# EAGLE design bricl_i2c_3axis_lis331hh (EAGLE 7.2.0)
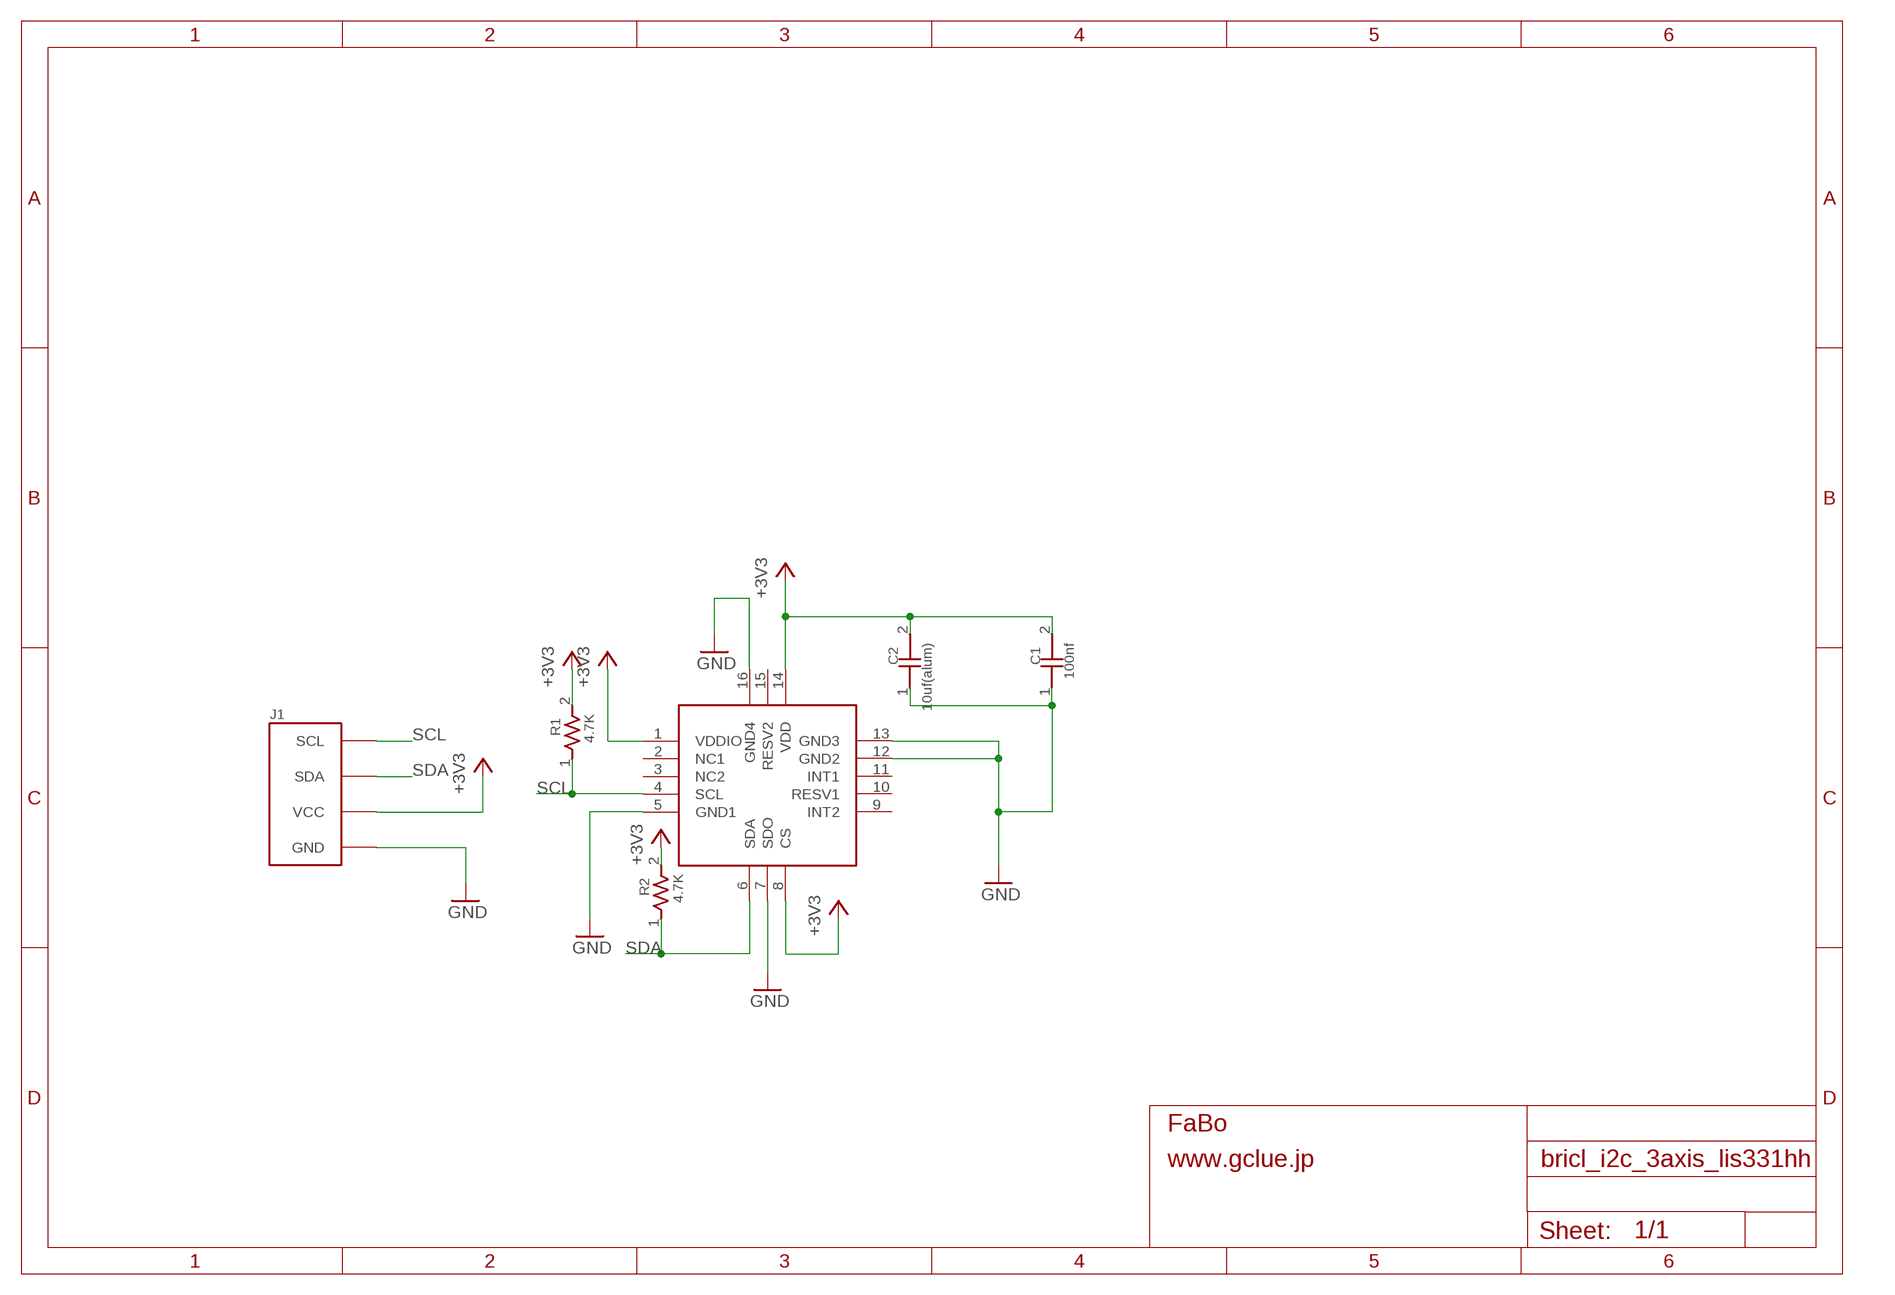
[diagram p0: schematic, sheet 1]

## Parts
C1  100nf  CAPACITOR0603  [0603]
C2  10uf(alum)  CAPACITOR0603  [0603]
J1  BRICK_I2C  [BRICK_I2C]
R1  4.7K  RESISTOR0603  [0603]
R2  4.7K  RESISTOR0603  [0603]
U$1  ST-LIS331HH  [ST-LIS331HH]

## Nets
+3V3: C1.2 C2.2 J1.VCC R1.2 R2.2 U$1.1(VDDIO) U$1.8(CS) U$1.14(VDD)
GND: C1.1 C2.1 J1.GND U$1.5(GND1) U$1.7(SDO) U$1.12(GND2) U$1.13(GND3) U$1.16(GND4)
SCL: J1.SCL R1.1 U$1.4(SCL)
SDA: J1.SDA R2.1 U$1.6(SDA)
Unconnected: U$1.2(NC1) U$1.3(NC2) U$1.9(INT2) U$1.10(RESV1) U$1.11(INT1) U$1.15(RESV2)

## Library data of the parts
C1 C2 = GClue-Capacitor:CAPACITOR
J1 = gclue:BRICK_I2C: FaBo Brick 4pin(I2C)
R1 R2 = GClue-Resistors:RESISTOR
U$1 = GClue-Mems:ST-LIS331HH

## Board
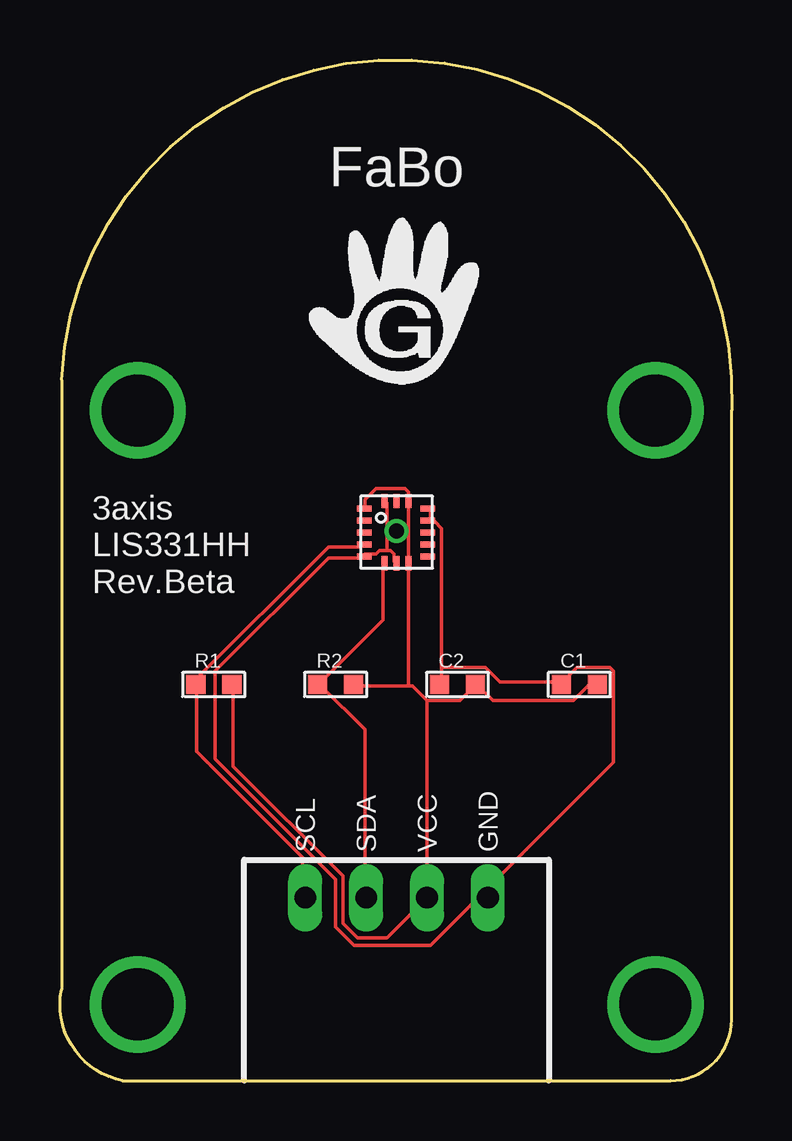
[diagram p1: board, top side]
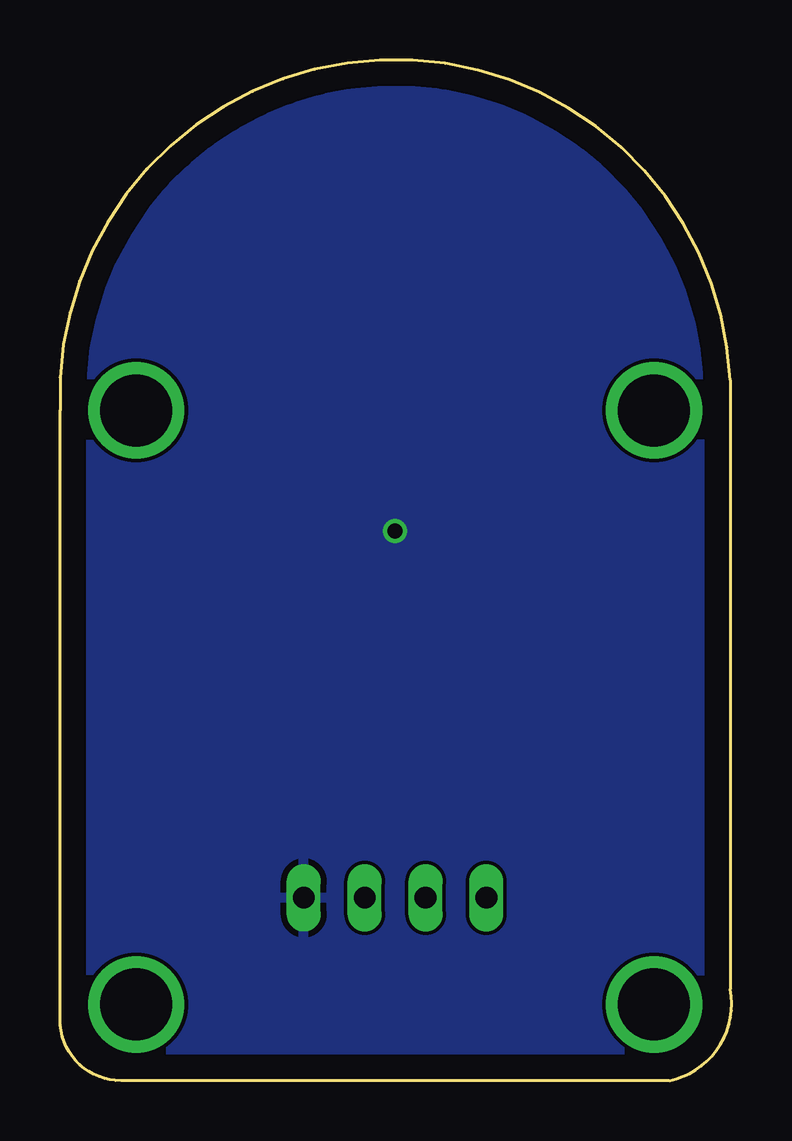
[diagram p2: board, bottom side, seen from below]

Size 28 x 42.55 mm. Coordinates in mm from the lower left corner, seen from the top.
Copper layers (1*16): Top 0.035mm / dielectric 1.5mm / Bottom 0.035mm
Design rules "default *": minimum track width 6mil, minimum drill 24mil, track to track 6mil, track to pad 6mil, pad to pad 6mil, via to via 6mil, smd to smd 6mil, copper to edge 40mil, drill to drill 8mil, minimum pad ring 10mil, minimum via ring 8mil, stop-mask expansion 4mil, vias tented up to drill 0mil, thermal gap 10mil

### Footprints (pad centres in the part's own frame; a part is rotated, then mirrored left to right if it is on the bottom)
0603 = smd 0.8 x 0.8: 1 -0.75,0; 2 0.75,0
BRICK_I2C = drill 0.9 long: GND 3.81,-12.7; SCL -3.81,-12.7; SDA -1.27,-12.7; VCC 1.27,-12.7 | drill 3 pad 3.81: P$5 -10.795,7.62; P$6 10.795,7.62; P$7 -10.795,-17.145; P$8 10.795,-17.145
ST-LIS331HH = smd 0.6 x 0.25: 1 -1.35,0.98; 2 -1.35,0.48; 3 -1.35,-0.02; 4 -1.35,-0.52; 5 -1.35,-1.02; 9 1.3,-1.02; 10 1.3,-0.52; 11 1.3,-0.02; 12 1.3,0.48; 13 1.3,0.98 | smd 0.25 x 0.6: 6 -0.5,-1.3; 7 0,-1.3; 8 0.5,-1.3; 14 0.5,1.3; 15 0,1.3; 16 -0.5,1.3

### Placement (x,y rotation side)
C1  21.65,16.51 0 top
C2  16.57,16.51 0 top
J1  14.03,20.32 0 top
R1  6.41,16.51 0 top
R2  11.49,16.51 0 top
U$1  14.03,22.86 0 top

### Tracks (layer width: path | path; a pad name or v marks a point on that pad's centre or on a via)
+3V3
  Top 0.152: U$1.1 12.71,23.93 12.71,24.23 13.17,24.69 14.39,24.69 14.54,24.54 14.54,24.23 U$1.14 14.54,24.08 14.54,21.64 U$1.8 14.54,21.49 14.54,16.46 | 14.54,16.46 14.69,16.46 15.3,15.85 | 14.54,16.46 12.25,16.46 R2.2 | 15.3,15.85 16.67,15.85 17.28,16.46 C2.2 17.44,16.46 18.05,15.85 21.4,15.85 22.01,16.46 22.31,16.46 C1.2 | R1.2 7.23,16.46 7.23,13.11 11.8,8.53 11.8,6.55 12.41,5.94 13.63,5.94 J1.VCC 15.3,15.85
GND  (via drill 0.61)
  Top 0.152: 13.63,22.1 13.78,22.1 13.93,21.95 13.93,21.64 U$1.7 | 13.63,22.1 13.32,22.1 13.17,21.95 12.71,21.95 U$1.5 12.56,21.79 11.19,21.79 6.46,17.07 6.46,13.41 11.49,8.38 11.49,6.4 12.25,5.64 15.45,5.64 23.07,13.26 23.07,17.07 22.92,17.22 21.55,17.22 20.94,16.61 C1.1 20.79,16.61 18.35,16.61 17.74,17.22 15.91,17.22 | 13.63,22.1 13.63,23.16 | 13.63,23.16 13.63,24.08 U$1.16 | v14.03,22.91 13.63,23.16 | 15.45,23.32 15.45,23.77 U$1.13 | 15.45,23.32 15.61,23.32 15.91,23.01 15.91,17.22 | 15.91,17.22 15.91,16.61 C2.1 | 15.45,23.32 U$1.12
  pour Bottom: 0.06,0 29.27,0 29.27,43.18 0.06,43.18
SCL
  Top 0.152: U$1.4 12.56,22.25 11.19,22.25 5.55,16.61 R1.1 5.7,16.46 5.7,13.72 10.12,9.3 10.12,7.62 J1.SCL
SDA
  Top 0.152: U$1.6 13.47,21.49 13.47,19.2 10.88,16.61 R2.1 10.88,16.46 12.71,14.63 12.71,7.62 J1.SDA

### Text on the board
tPlace: 3axis / LIS331HH / Rev.Beta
